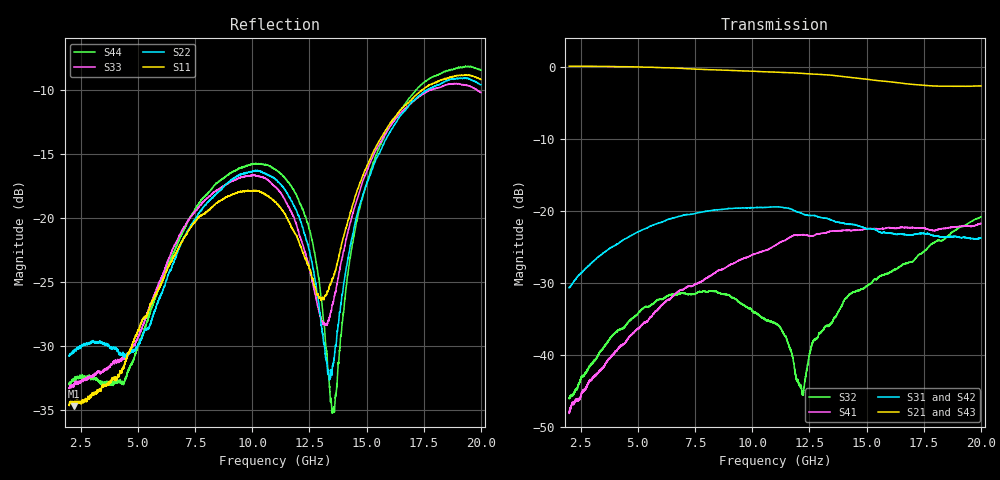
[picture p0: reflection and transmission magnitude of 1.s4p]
!Keysight Technologies,N5225A,MY51451420,A.10.40.12
!Date: Thursday, October 15, 2015 10:55:23
!Correction: S11(Full 4 Port(1,2,3,4))
!S12(Full 4 Port(1,2,3,4))
!S13(Full 4 Port(1,2,3,4))
!S14(Full 4 Port(1,2,3,4))
!S21(Full 4 Port(1,2,3,4))
!S22(Full 4 Port(1,2,3,4))
!S23(Full 4 Port(1,2,3,4))
!S24(Full 4 Port(1,2,3,4))
!S31(Full 4 Port(1,2,3,4))
!S32(Full 4 Port(1,2,3,4))
!S33(Full 4 Port(1,2,3,4))
!S34(Full 4 Port(1,2,3,4))
!S41(Full 4 Port(1,2,3,4))
!S42(Full 4 Port(1,2,3,4))
!S43(Full 4 Port(1,2,3,4))
!S44(Full 4 Port(1,2,3,4))
!S4P File: Measurements: <S11,S12,S13,S14>,
!<S21,S22,S23,S24>,
!<S31,S32,S33,S34>,
!<S41,S42,S43,S44>:
# Hz S  dB  R 50
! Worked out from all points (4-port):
!   6401 points, 2 GHz to 20 GHz, reference 50 ohm
!   strongest paths, dB at 2 GHz, 6.5 GHz, 11 GHz, 15.5 GHz, 20 GHz:
!     S21: 0.1, -0.2, -0.7, -1.9, -2.6
!     S43: 0.0, -0.2, -0.8, -2.0, -2.7
!     S31: -30.7, -21.0, -19.5, -22.8, -23.8
!     S42: -30.8, -21.1, -19.5, -22.8, -23.9
!     S41: -48.1, -32.0, -24.8, -22.5, -21.7
!     S32: -46.1, -31.6, -35.7, -29.3, -20.9
!   lowest |S11| = -34.7 dB at 2.219 GHz (marker M1), VSWR 1.04, Z = 49.2 + j1.62 ohm
!   |S11| at or under -10 dB: start of sweep to 17.42 GHz; 17.42229 GHz to 17.42412 GHz (1.831 MHz wide, 0.0105 % of centre)
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2e9  -34.67 119.2  0.09 -35.7  -30.69 53.6  -48.00 46.8
     0.09 -35.7  -30.77 57.3  -46.06 84.3  -30.72 53.5
     -30.69 53.5  -46.08 85.3  -33.31 41.2  -0.00 -36.1
     -48.14 46.0  -30.76 53.6  -0.01 -36.1  -33.04 71.2
2.219375e9  -34.75 116.0  0.08 -39.6  -29.76 50.2  -46.66 35.6
            0.09 -39.6  -30.40 49.4  -45.32 80.9  -29.87 50.3
            -29.76 50.3  -45.38 80.7  -32.98 34.4  -0.01 -40.0
            -46.63 35.6  -29.86 50.4  -0.01 -40.1  -32.66 68.6
5.653438e9  -26.44 123.3  -0.07 -101.6  -22.00 -14.1  -34.50 -56.8
            -0.07 -101.7  -27.73 -127.6  -32.94 7.4  -22.12 -13.9
            -22.01 -14.1  -32.94 7.5  -26.34 -139.9  -0.15 -102.8
            -34.45 -56.7  -22.13 -13.9  -0.15 -102.8  -26.81 114.2
9.844062e9  -17.86 54.4  -0.59 -177.6  -19.59 -97.0  -26.36 -176.8
            -0.59 -177.7  -16.40 96.1  -33.59 -98.5  -19.69 -97.3
            -19.58 -97.0  -33.54 -98.4  -16.71 91.1  -0.68 -179.7
            -26.38 -176.9  -19.69 -97.3  -0.68 -179.7  -15.85 60.0
1.354531e10  -24.69 -142.7  -1.19 112.4  -21.40 -167.5  -22.80 88.8
             -1.19 112.3  -31.44 -100.0  -35.18 -78.8  -21.44 -168.3
             -21.39 -167.6  -35.17 -78.3  -26.63 -122.1  -1.25 109.7
             -22.79 88.6  -21.44 -168.3  -1.27 109.6  -35.13 -117.0
1.555906e10  -13.97 136.8  -1.94 74.5  -22.92 163.3  -22.53 44.8
             -1.94 74.4  -14.99 154.8  -29.16 -116.7  -22.94 160.7
             -22.93 163.3  -29.12 -116.3  -14.24 152.6  -2.02 71.3
             -22.52 44.7  -22.92 160.7  -2.02 71.2  -14.52 129.5
2e10  -9.15 33.9  -2.65 -7.9  -23.81 95.4  -21.75 -29.1
      -2.65 -8.1  -9.57 60.0  -20.88 141.6  -23.86 95.3
      -23.78 95.5  -20.85 141.7  -10.18 54.9  -2.64 -11.9
      -21.75 -29.3  -23.86 95.3  -2.65 -11.9  -8.43 38.4
